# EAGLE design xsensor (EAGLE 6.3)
FrSky SPORT adapter for rpm
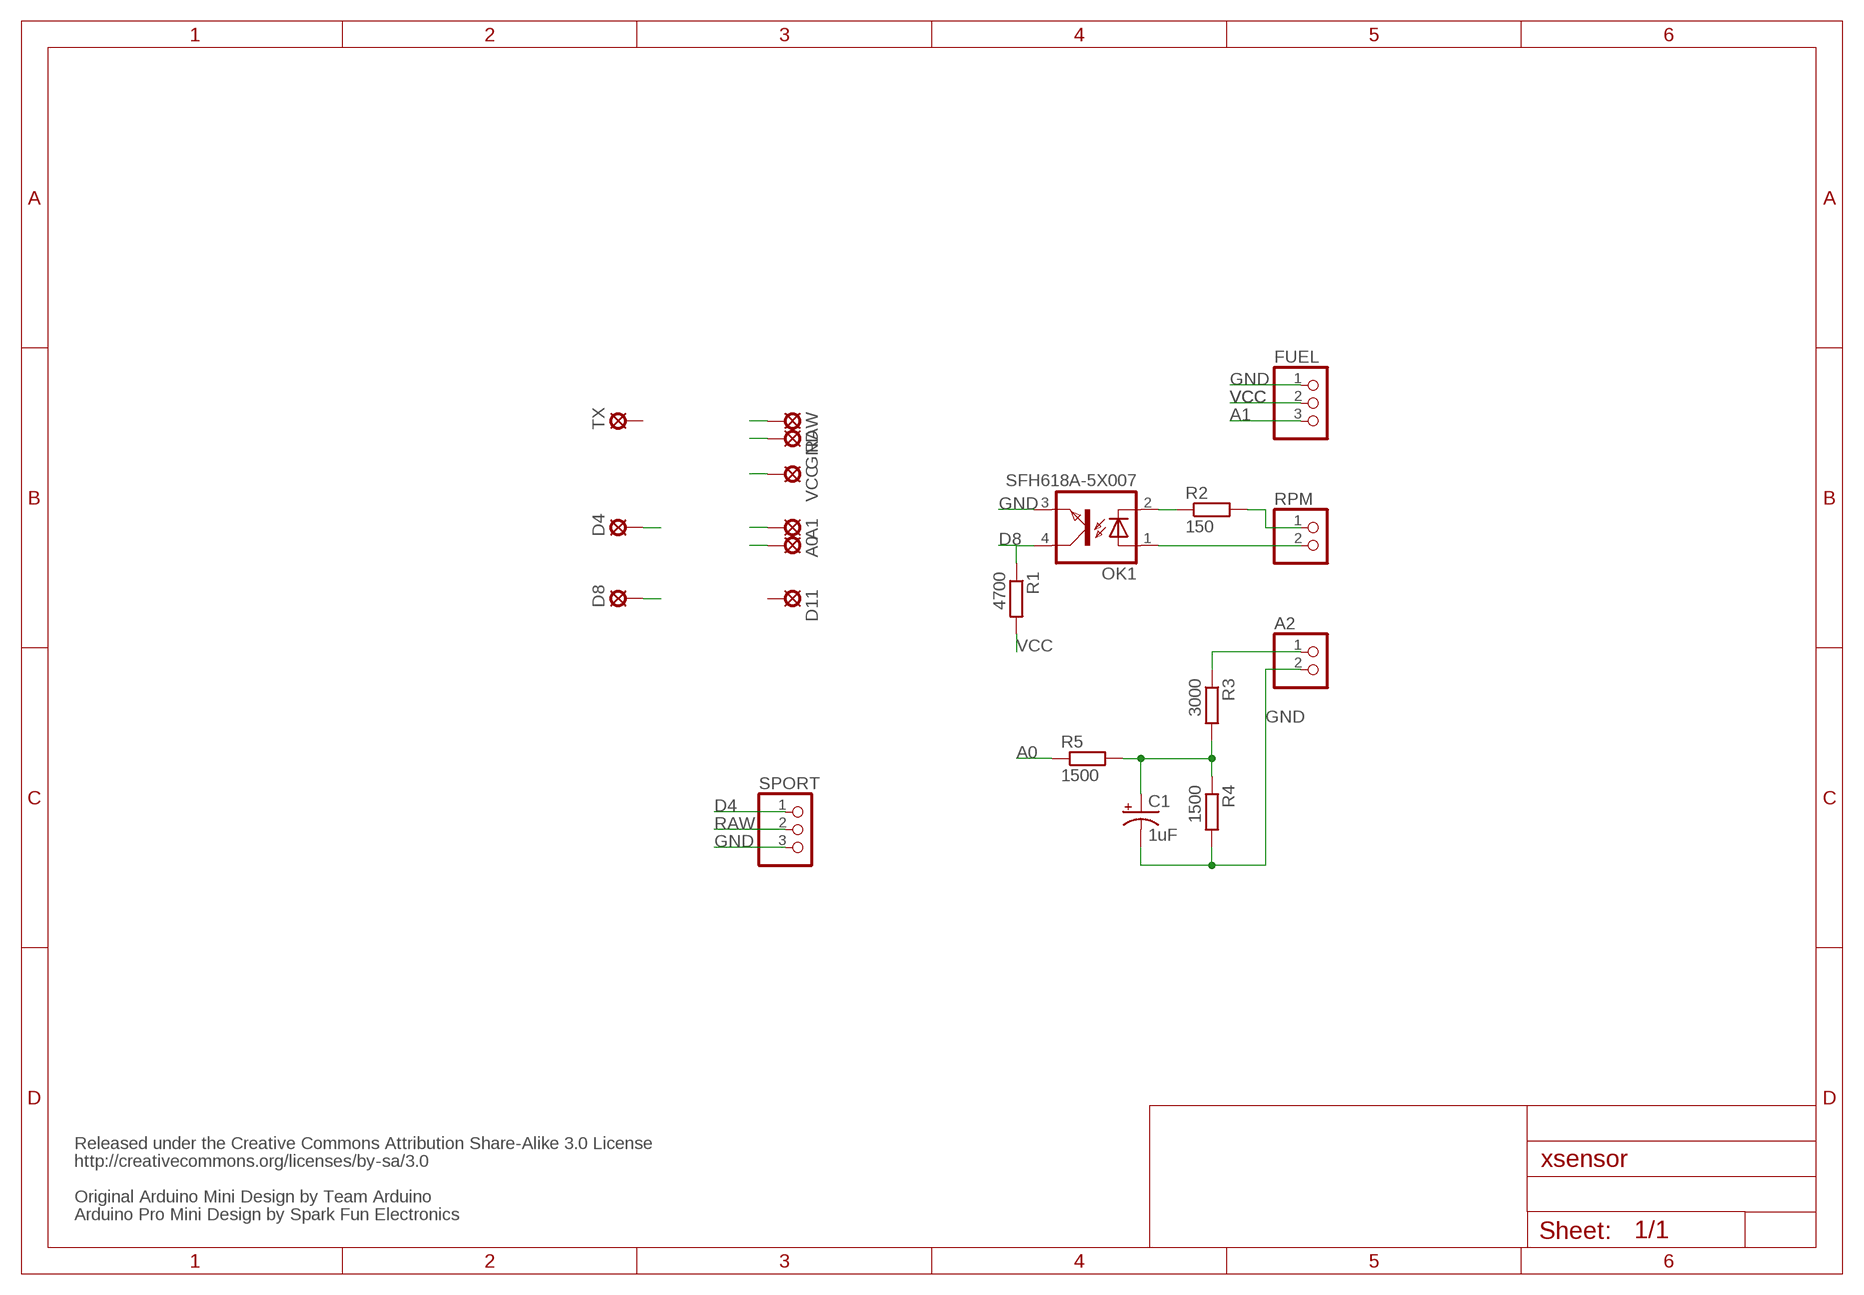
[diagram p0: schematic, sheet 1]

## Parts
A0  LSP10  [LSP10]
A1  LSP10  [LSP10]
A2  PINHD-1X2  [1X02]
C1  1uF  CPOL-USB/3528-21R  [B/3528-21R]
D4  LSP10  [LSP10]
D8  LSP10  [LSP10]
D11  LSP10  [LSP10]
FUEL  PINHD-1X3  [1X03]
GND  LSP10  [LSP10]
OK1  SFH618A-5X007  [SMD4-7]
R1  4700  R-EU_0204/7  [0204/7]
R2  150  R-EU_R1206  [R1206]
R3  3000  R-EU_R1206  [R1206]
R4  1500  R-EU_R1206  [R1206]
R5  1500  R-EU_R1206  [R1206]
RAW  LSP10  [LSP10]
RPM  PINHD-1X2  [1X02]
SPORT  PINHD-1X3/90  [1X03/90]
TX  LSP10  [LSP10]
VCC  LSP10  [LSP10]

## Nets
A0: A0.MP R5.1
A1: A1.MP FUEL.3
D4: D4.MP SPORT.1
D8: D8.MP OK1.4(COL) R1.1
GND [vcc]: A2.2 C1.- FUEL.1 GND.MP OK1.3(EMIT) R4.2 SPORT.3
N$4: OK1.2(C) R2.1
N$5: R2.2 RPM.1
N$6: OK1.1(A) RPM.2
N$8: A2.1 R3.1
RAW [vcc]: RAW.MP SPORT.2
VCC: FUEL.2 R1.2 VCC.MP
VPART: C1.+ R3.2 R4.1 R5.2
Unconnected: D11.MP TX.MP

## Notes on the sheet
- Released under the Creative Commons Attribution Share-Alike 3.0 License
- http://creativecommons.org/licenses/by-sa/3.0
- Original Arduino Mini Design by Team Arduino
- Arduino Pro Mini Design by Spark Fun Electronics

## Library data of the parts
A0 A1 D4 D8 D11 GND RAW TX VCC = solpad:LSP10: SOLDER PAD
A2 RPM = pinhead:PINHD-1X2: PIN HEADER
C1 = rcl:CPOL-US: POLARIZED CAPACITOR, American symbol
FUEL SPORT = pinhead:PINHD-1X3: PIN HEADER
OK1 = optocoupler:SFH618?*: Optocoupler, Phototransistor Output, Low Input Current Source: Data sheet; MPN: SFH618A-5X007; OC_FARNELL: unknown; OC_NEWARK: 43K9546
R1-R5 = resistor:R-EU_: RESISTOR, European symbol

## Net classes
0 default: width 0.203 mm
1 vcc: width 0.254 mm

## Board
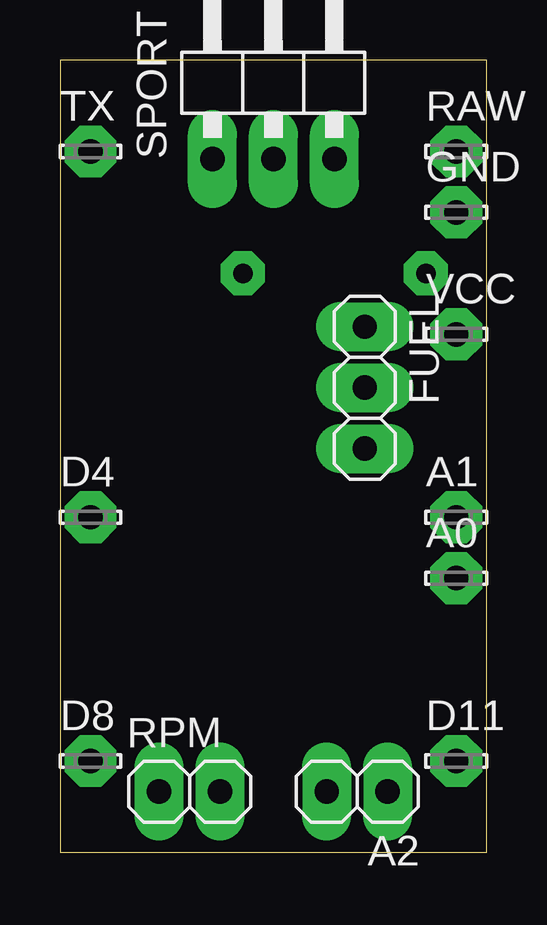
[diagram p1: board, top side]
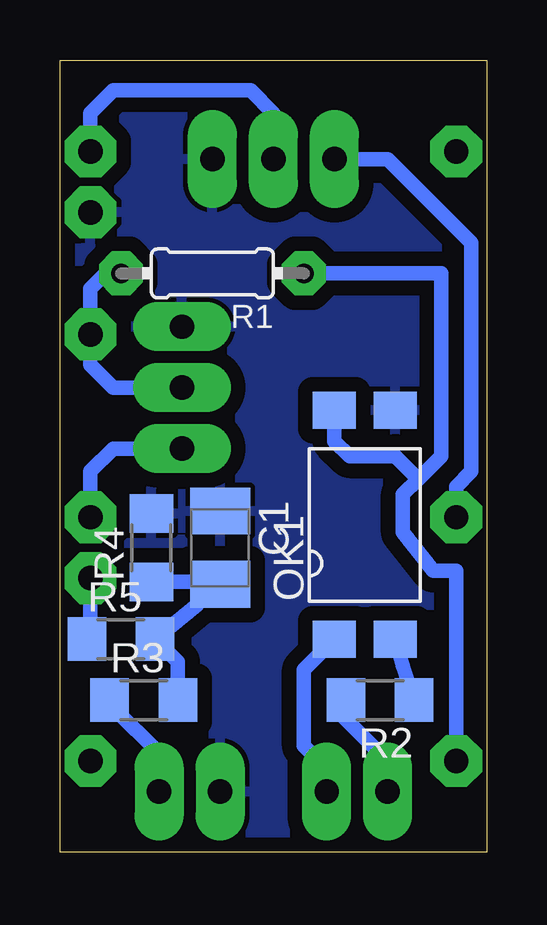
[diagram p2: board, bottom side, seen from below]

Size 17.78 x 33.02 mm. Coordinates in mm from the lower left corner, seen from the top.
Outline: 0,33.02 0,0 17.78,0 17.78,33.02 0,33.02
Copper layers (1*16): Top 0.035mm / dielectric 1.5mm / Bottom 0.035mm
Design rules "romolo *": minimum track width 16mil, minimum drill 16mil, track to track 8mil, track to pad 8mil, pad to pad 8mil, via to via 8mil, smd to smd 8mil, copper to edge 8mil, drill to drill 8mil, minimum pad ring 20mil, minimum via ring 8mil, stop-mask expansion 4mil, vias tented up to drill 0mil, thermal gap 8mil

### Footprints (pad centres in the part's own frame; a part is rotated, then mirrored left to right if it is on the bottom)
LSP10 = drill 1.016 pad 2.159 octagon: MP 0,0
1X02 = drill 1.016 long: 1 -1.27,0; 2 1.27,0
B/3528-21R = smd 1.95 x 2.5: + 1.525,0; - -1.525,0
1X03 = drill 1.016 long: 1 -2.54,0; 2 0,0; 3 2.54,0
SMD4-7 = smd 1.78 x 1.55: 1 -1.27,-4.77; 2 1.27,-4.77; 3 1.27,4.77; 4 -1.27,4.77
0204/7 = drill 0.813 octagon: 1 -3.81,0; 2 3.81,0
R1206 = smd 1.6 x 1.803: 1 -1.422,0; 2 1.422,0
1X03/90 = drill 1.016 long: 1 -2.54,-3.81; 2 0,-3.81; 3 2.54,-3.81

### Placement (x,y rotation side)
A0  16.51,11.43 0 top
A1  16.51,13.97 0 top
A2  12.38,2.54 180 top
C1  11.11,12.7 270 bottom
D4  1.27,13.97 0 top
D8  1.27,3.81 0 top
D11  16.51,3.81 0 top
FUEL  12.7,19.37 270 top
GND  16.51,26.67 0 top
OK1  5.08,13.65 0 bottom
R1  11.43,24.13 180 bottom
R2  4.45,6.35 180 bottom
R3  14.29,6.35 0 bottom
R4  13.97,12.7 90 bottom
R5  15.24,8.89 0 bottom
RAW  16.51,29.21 0 top
RPM  5.4,2.54 0 top
SPORT  8.89,32.7 0 top
TX  1.27,29.21 0 top
VCC  16.51,21.59 0 top

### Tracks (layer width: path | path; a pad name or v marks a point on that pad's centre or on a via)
A0
  Bottom 0.61: A0.MP 16.51,8.89 R5.1
A1
  Bottom 0.61: FUEL.3 15.56,16.83 16.51,15.88 A1.MP
D4
  Bottom 0.61: D4.MP 1.27,15.24 0.64,15.88 0.64,25.4 4.13,28.89 SPORT.1
D8
  Bottom 0.61: R1.1 1.91,24.13 1.91,16.51 2.86,15.56 | OK1.4 6.35,17.14 5.71,16.51 3.81,16.51 2.86,15.56 | D8.MP 1.27,11.75 2.22,11.75 3.49,13.34 3.49,14.92 2.86,15.56
GND
  pour Bottom (isolate 0.61): 0,33.02 17.78,33.02 17.78,0 0,0
N$4
  Bottom 0.61: R2.1 3.49,7.77 OK1.2
N$5
  Bottom 0.61: RPM.1 4.13,3.81 6.03,5.71 6.03,6.2 R2.2
N$6
  Bottom 0.61: RPM.2 6.67,3.49 7.62,4.45 7.62,7.61 OK1.1
N$8
  Bottom 0.61: R3.1 15.56,6.83 15.56,6.03 13.65,4.13 A2.1
RAW
  Bottom 0.61: SPORT.2 8.89,30.8 9.84,31.75 15.56,31.75 16.51,30.8 RAW.MP
VCC
  Bottom 0.61: FUEL.2 15.56,19.37 16.51,20.32 VCC.MP 16.51,23.5 15.88,24.13 R1.2
VPART
  Bottom 0.61: C1.+ 10.5,10.96 10.82,11.28 12.06,11.28 | 12.06,11.28 R4.1 | 12.06,11.28 12.06,10.31 R5.2 12.87,7.94 R3.2

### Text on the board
tValues: Tent Vias! | Arduino Wee v1.3
tTest: S/PORT | TX | - | FUEL | RPM | - | - | A2 | D11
